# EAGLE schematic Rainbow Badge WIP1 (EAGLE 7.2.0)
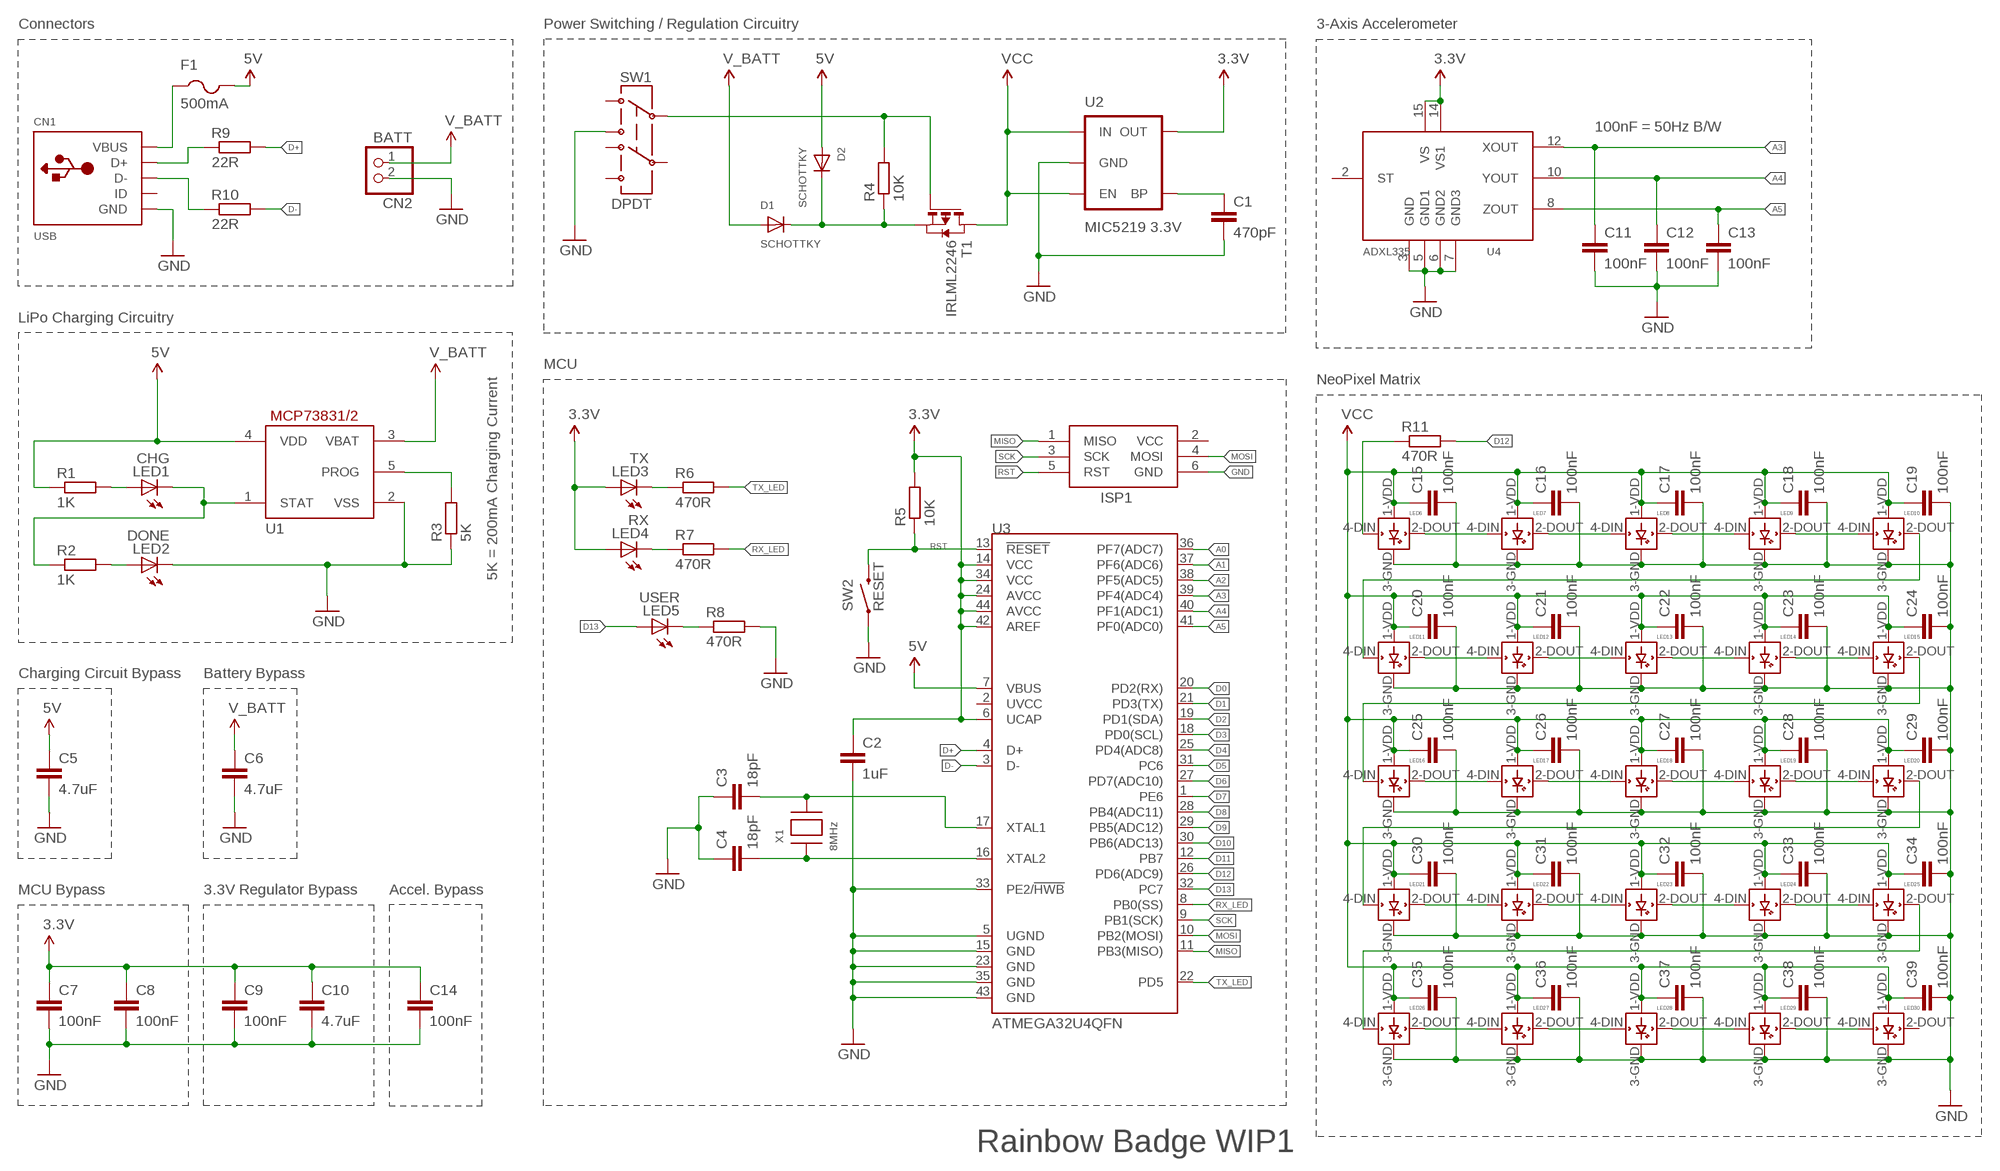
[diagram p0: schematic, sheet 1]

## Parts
C1  470pF  C-EUC0603  [C0603]
C2  1uF  C-EUC0603  [C0603]
C3  18pF  C-EUC0603  [C0603]
C4  18pF  C-EUC0603  [C0603]
C5  4.7uF  C-EUC1206  [C1206]
C6  4.7uF  C-EUC1206  [C1206]
C7  100nF  C-EUC0603  [C0603]
C8  100nF  C-EUC0603  [C0603]
C9  100nF  C-EUC0603  [C0603]
C10  4.7uF  C-EUC0603  [C0603]
C11  100nF  C-EUC0603  [C0603]
C12  100nF  C-EUC0603  [C0603]
C13  100nF  C-EUC0603  [C0603]
C14  100nF  C-EUC0603  [C0603]
C15  100nF  C-EUC0805  [C0805]
C16  100nF  C-EUC0805  [C0805]
C17  100nF  C-EUC0805  [C0805]
C18  100nF  C-EUC0805  [C0805]
C19  100nF  C-EUC0805  [C0805]
C20  100nF  C-EUC0805  [C0805]
C21  100nF  C-EUC0805  [C0805]
C22  100nF  C-EUC0805  [C0805]
C23  100nF  C-EUC0805  [C0805]
C24  100nF  C-EUC0805  [C0805]
C25  100nF  C-EUC0805  [C0805]
C26  100nF  C-EUC0805  [C0805]
C27  100nF  C-EUC0805  [C0805]
C28  100nF  C-EUC0805  [C0805]
C29  100nF  C-EUC0805  [C0805]
C30  100nF  C-EUC0805  [C0805]
C31  100nF  C-EUC0805  [C0805]
C32  100nF  C-EUC0805  [C0805]
C33  100nF  C-EUC0805  [C0805]
C34  100nF  C-EUC0805  [C0805]
C35  100nF  C-EUC0805  [C0805]
C36  100nF  C-EUC0805  [C0805]
C37  100nF  C-EUC0805  [C0805]
C38  100nF  C-EUC0805  [C0805]
C39  100nF  C-EUC0805  [C0805]
CN1  USB  USBMINIB  [USB-MINIB]
CN2  BATT  JST_2PIN-SMT-RA  [JST-PH-2-SMT-RA]
D1  SCHOTTKY  DIODESOD-123  [SOD-123]
D2  SCHOTTKY  DIODESOD-123  [SOD-123]
F1  500mA  PTCFUSE-1206  [R1206]
ISP1  AVRISP  AVRISP-6  [AVRISP]
LED1  CHG  LEDCHIP-LED0603  [CHIP-LED0603]
LED2  DONE  LEDCHIP-LED0603  [CHIP-LED0603]
LED3  TX  LEDCHIP-LED0603  [CHIP-LED0603]
LED4  RX  LEDCHIP-LED0603  [CHIP-LED0603]
LED5  USER  LEDCHIP-LED0603  [CHIP-LED0603]
LED6  WS2812B  [WS2812B]
LED7  WS2812B  [WS2812B]
LED8  WS2812B  [WS2812B]
LED9  WS2812B  [WS2812B]
LED10  WS2812B  [WS2812B]
LED11  WS2812B  [WS2812B]
LED12  WS2812B  [WS2812B]
LED13  WS2812B  [WS2812B]
LED14  WS2812B  [WS2812B]
LED15  WS2812B  [WS2812B]
LED16  WS2812B  [WS2812B]
LED17  WS2812B  [WS2812B]
LED18  WS2812B  [WS2812B]
LED19  WS2812B  [WS2812B]
LED20  WS2812B  [WS2812B]
LED21  WS2812B  [WS2812B]
LED22  WS2812B  [WS2812B]
LED23  WS2812B  [WS2812B]
LED24  WS2812B  [WS2812B]
LED25  WS2812B  [WS2812B]
LED26  WS2812B  [WS2812B]
LED27  WS2812B  [WS2812B]
LED28  WS2812B  [WS2812B]
LED29  WS2812B  [WS2812B]
LED30  WS2812B  [WS2812B]
R1  1K  R-EU_R0603  [R0603]
R2  1K  R-EU_R0603  [R0603]
R3  5K  R-EU_R0603  [R0603]
R4  10K  R-EU_R0603  [R0603]
R5  10K  R-EU_R0603  [R0603]
R6  470R  R-EU_R0603  [R0603]
R7  470R  R-EU_R0603  [R0603]
R8  470R  R-EU_R0603  [R0603]
R9  22R  R-EU_R0603  [R0603]
R10  22R  R-EU_R0603  [R0603]
R11  470R  R-EU_R0603  [R0603]
SW1  DPDT  SWITCH-DPDTAYZ0202  [AYZ0202]
SW2  RESET  SWITCH-MOMENTARY-2SMD  [TACTILE-SWITCH-SMD]
T1  IRLML2246  PMOSSOT23  [SOT-23]
U1  MCP73831/OT  [SOT23-5L]
U2  MIC5219 3.3V  V_REG_MIC52193.3V  [SOT23-5]
U3  ATMEGA32U4QFN  [QFN-44]
U4  ADXL335  ADXL33X  [16LCSP]
X1  8MHz  XTALNX5032  [NX5032]

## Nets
3.3V: C2.1 C7.1 C8.1 C9.1 C10.1 C14.1 LED3.A LED4.A R5.2 U2.5(OUT) U3.6(UCAP) U3.14(VCC) U3.24(AVCC) U3.34(VCC) U3.42(AREF) U3.44(AVCC) U4.14(VS1) U4.15(VS)
5V: C5.1 D2.A F1.2 R1.1 U1.4(VDD) U3.7(VBUS)
A0: U3.36(PF7(ADC7))
A1: U3.37(PF6(ADC6))
A2: U3.38(PF5(ADC5))
A3: C11.1 U3.39(PF4(ADC4)) U4.12(XOUT)
A4: C12.1 U3.40(PF1(ADC1)) U4.10(YOUT)
A5: C13.1 U3.41(PF0(ADC0)) U4.8(ZOUT)
D0: U3.20(PD2(RX))
D1: U3.21(PD3(TX))
D2: U3.19(PD1(SDA))
D3: U3.18(PD0(SCL))
D4: U3.25(PD4(ADC8))
D5: U3.31(PC6)
D6: U3.27(PD7(ADC10))
D7: U3.1(PE6)
D8: U3.28(PB4(ADC11))
D9: U3.29(PB5(ADC12))
D10: U3.30(PB6(ADC13))
D11: U3.12(PB7)
D12: R11.2 U3.26(PD6(ADC9))
D13: LED5.A U3.32(PC7)
D+: R9.2 U3.4(D+)
D-: R10.2 U3.3(D-)
GND: C1.2 C2.2 C3.1 C4.1 C5.2 C6.2 C7.2 C8.2 C9.2 C10.2 C11.2 C12.2 C13.2 C14.2 C15.2 C16.2 C17.2 C18.2 C19.2 C20.2 C21.2 C22.2 C23.2 C24.2 C25.2 C26.2 C27.2 C28.2 C29.2 C30.2 C31.2 C32.2 C33.2 C34.2 C35.2 C36.2 C37.2 C38.2 C39.2 CN1.GND CN2.2 ISP1.6(GND) LED2.C LED6.3-GND(GND) LED7.3-GND(GND) LED8.3-GND(GND) LED9.3-GND(GND) LED10.3-GND(GND) LED11.3-GND(GND) LED12.3-GND(GND) LED13.3-GND(GND) LED14.3-GND(GND) LED15.3-GND(GND) LED16.3-GND(GND) LED17.3-GND(GND) LED18.3-GND(GND) LED19.3-GND(GND) LED20.3-GND(GND) LED21.3-GND(GND) LED22.3-GND(GND) LED23.3-GND(GND) LED24.3-GND(GND) LED25.3-GND(GND) LED26.3-GND(GND) LED27.3-GND(GND) LED28.3-GND(GND) LED29.3-GND(GND) LED30.3-GND(GND) R3.1 R8.2 SW1.3 SW2.1 U1.2(VSS) U2.2(GND) U3.5(UGND) U3.15(GND) U3.23(GND) U3.33(PE2/!HWB) U3.35(GND) U3.43(GND) U4.3(GND) U4.5(GND1) U4.6(GND2) U4.7(GND3)
MISO: ISP1.1(MISO) U3.11(PB3(MISO))
MOSI: ISP1.4(MOSI) U3.10(PB2(MOSI))
N$1: LED1.C R2.1 U1.1(STAT)
N$2: LED2.A R2.2
N$3: LED1.A R1.2
N$4: R3.2 U1.5(PROG)
N$5: CN1.VBUS F1.1
N$6: LED3.C R6.1
N$7: C1.1 U2.4(BP)
N$8: R4.2 SW1.2 T1.3(G)
N$9: D1.C D2.C R4.1 T1.2(S)
N$10: C3.2 U3.17(XTAL1) X1.P$2
N$11: C4.2 U3.16(XTAL2) X1.P$1
N$12: LED4.C R7.1
N$13: LED5.C R8.1
N$14: CN1.D+ R9.1
N$15: CN1.D- R10.1
N$16: LED6.4-DIN(DIN) R11.1
N$66: LED6.2-DOUT(DOUT) LED7.4-DIN(DIN)
N$67: LED7.2-DOUT(DOUT) LED8.4-DIN(DIN)
N$68: LED8.2-DOUT(DOUT) LED9.4-DIN(DIN)
N$69: LED9.2-DOUT(DOUT) LED10.4-DIN(DIN)
N$70: LED11.2-DOUT(DOUT) LED12.4-DIN(DIN)
N$71: LED12.2-DOUT(DOUT) LED13.4-DIN(DIN)
N$72: LED13.2-DOUT(DOUT) LED14.4-DIN(DIN)
N$73: LED14.2-DOUT(DOUT) LED15.4-DIN(DIN)
N$74: LED16.2-DOUT(DOUT) LED17.4-DIN(DIN)
N$75: LED17.2-DOUT(DOUT) LED18.4-DIN(DIN)
N$76: LED18.2-DOUT(DOUT) LED19.4-DIN(DIN)
N$77: LED19.2-DOUT(DOUT) LED20.4-DIN(DIN)
N$78: LED21.2-DOUT(DOUT) LED22.4-DIN(DIN)
N$79: LED22.2-DOUT(DOUT) LED23.4-DIN(DIN)
N$80: LED23.2-DOUT(DOUT) LED24.4-DIN(DIN)
N$81: LED24.2-DOUT(DOUT) LED25.4-DIN(DIN)
N$82: LED26.2-DOUT(DOUT) LED27.4-DIN(DIN)
N$83: LED27.2-DOUT(DOUT) LED28.4-DIN(DIN)
N$84: LED28.2-DOUT(DOUT) LED29.4-DIN(DIN)
N$85: LED29.2-DOUT(DOUT) LED30.4-DIN(DIN)
N$86: LED10.2-DOUT(DOUT) LED11.4-DIN(DIN)
N$87: LED15.2-DOUT(DOUT) LED16.4-DIN(DIN)
N$88: LED20.2-DOUT(DOUT) LED21.4-DIN(DIN)
N$89: LED25.2-DOUT(DOUT) LED26.4-DIN(DIN)
RST: ISP1.5(RST) R5.1 SW2.3 U3.13(!RESET)
RX_LED: R7.2 U3.8(PB0(SS))
SCK: ISP1.3(SCK) U3.9(PB1(SCK))
TX_LED: R6.2 U3.22(PD5)
V_BATT: C6.1 CN2.1 D1.A U1.3(VBAT)
VCC: C15.1 C16.1 C17.1 C18.1 C19.1 C20.1 C21.1 C22.1 C23.1 C24.1 C25.1 C26.1 C27.1 C28.1 C29.1 C30.1 C31.1 C32.1 C33.1 C34.1 C35.1 C36.1 C37.1 C38.1 C39.1 LED6.1-VDD(VDD) LED7.1-VDD(VDD) LED8.1-VDD(VDD) LED9.1-VDD(VDD) LED10.1-VDD(VDD) LED11.1-VDD(VDD) LED12.1-VDD(VDD) LED13.1-VDD(VDD) LED14.1-VDD(VDD) LED15.1-VDD(VDD) LED16.1-VDD(VDD) LED17.1-VDD(VDD) LED18.1-VDD(VDD) LED19.1-VDD(VDD) LED20.1-VDD(VDD) LED21.1-VDD(VDD) LED22.1-VDD(VDD) LED23.1-VDD(VDD) LED24.1-VDD(VDD) LED25.1-VDD(VDD) LED26.1-VDD(VDD) LED27.1-VDD(VDD) LED28.1-VDD(VDD) LED29.1-VDD(VDD) LED30.1-VDD(VDD) T1.1(D) U2.1(IN) U2.3(EN)
Unconnected: CN1.ID LED30.2-DOUT(DOUT) SW1.1 SW1.4 SW1.5 SW1.6 U3.2(UVCC) U4.2(ST)

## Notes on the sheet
- Connectors | Power Switching / Regulation Circuitry | 3-Axis Accelerometer
- 100nF = 50Hz B/W
- LiPo Charging Circuitry
- MCU
- NeoPixel Matrix
- 5K = 200mA Charging Current
- Charging Circuit Bypass | Battery Bypass
- MCU Bypass | 3.3V Regulator Bypass | Accel. Bypass
- Rainbow Badge WIP1

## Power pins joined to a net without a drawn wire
VCC: ISP1.2(VCC)

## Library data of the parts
C1-C39 = rcl:C-EU: CAPACITOR, European symbol
CN1 = adafruit:USB: USB Connectors USBMINIB - Surface Mount Female Mini-B USB Connector 4UConnector: 06564 By microbuilder.eu Thru-hole RA Female Mini-B USB Connector 4UConnector: 18732 By ladyada.net
CN2 = adafruit:JST_2PIN: JST 2-Pin Connectors of various flavors
D1 D2 = adafruit:DIODE: Diode
F1 = adafruit:PTCFUSE: PTC fuses, resettable thermistors
ISP1 = adafruit:AVRISP: AVR ISP HEADER Standard 6 pin header for AVR programming
LED1-LED5 = led:LED: LED
LED6-LED30 = adafruit:WS2812B
R1-R11 = rcl:R-EU_: RESISTOR, European symbol
SW1 = SparkFun-Electromechanical:SWITCH-DPDT: DPDT Version of the COM-00597; PROD_ID: SWCH-08179
SW2 = SparkFun-Electromechanical:SWITCH-MOMENTARY-2: Various NO switches- pushbuttons, reed, etc; PROD_ID: SWCH-08247
T1 = zetex:PMOSSOT23: MOS FET; OC_FARNELL: unknown; OC_NEWARK: unknown
U1 = adafruit:MCP73831: MCP73831/2 Miniature Single-Cell, Fully Integrated Li-Ion, Li-Polymer Charge Management Controllers. Nice and small simple lipoly charge controller, with adjustable current and status output (LED) http://www.ladyada.net/library/pcb/eaglelibrary.html
U2 = SparkFun-PowerIC:V_REG_MIC5219: V_REG MIC5219 Standard 3.3V and 5V 500mA LDO voltage regulator in SOT-23 layout. Micrel part MIC5219. BP (by-pass) pin is used to lower output noise with 470pF cap, may be left open.; PROD_ID: VREG-09872
U3 = SparkFun-DigitalIC:ATMEGA32U4: Atmel 44-pin 8-bit Microcontroller with 32KBytes of ISP Flash and USB Controller
U4 = adafruit:ADXL33X
X1 = adafruit:XTAL: Low cost SMT crystals, no capacitors included

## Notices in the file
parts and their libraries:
SparkFun-Aesthetics: Licensing: Creative Commons ShareAlike 4.0 International - https://creativecommons.org/licenses/by-sa/4.0
